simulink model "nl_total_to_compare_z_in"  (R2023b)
settings: Solver=VariableStepAuto  StartTime=0  StopTime=t(end)  RelTol=1e-9  AbsTol=1e-9
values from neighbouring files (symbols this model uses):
  cp_H2_coeff = [a_H2 b_H2 c_H2 d_H2]    [run_connect_all_sELY.m]
  cp_O2_coeff = [a_O2 b_O2 c_O2 d_O2]    [run_connect_all_sELY.m]
  eta_ACDC = 0.95    [run_connect_all_sELY.m]
  f1 = deg_model_eMTI.f1    [run_connect_all_sELY.m]
  f2 = deg_model_eMTI.f2    [run_connect_all_sELY.m]
  f3 = deg_model_eMTI.f3    [run_connect_all_sELY.m]
  f4 = deg_model_eMTI.f4    [run_connect_all_sELY.m]
  f5 = deg_model_eMTI.f5    [run_connect_all_sELY.m]
  F_farad = 96485    [run_connect_all_sELY.m]
  K_AW = 1/K_P    (= 2e-05)    [run_connect_all_sELY.m]
  K_I = 500    [run_connect_all_sELY.m]
  K_Ic = 0.01    [run_connect_all_sELY.m]
  K_max = P_cool_lim    (= 350000)    [run_connect_all_sELY.m]
  K_min = 0    [run_connect_all_sELY.m]
  K_P = 50000    [run_connect_all_sELY.m]
  M_H2 = 2.0159*1e-3    (= 0.0020159)    [run_connect_all_sELY.m]
  p_an = 29    [run_connect_all_sELY.m]
  p_BoP_prod = 0.05    [run_connect_all_sELY.m]
  P_BoP_sb = 7.1258e+03    (= 7125.8)    [run_connect_all_sELY.m]
  p_cat = 30    [run_connect_all_sELY.m]
  P_min_solve = 1e-3    (= 0.001)    [run_connect_all_sELY.m]
  R = 8.3145    [run_connect_all_sELY.m]    (also in DemoMTI_DHN_Pongau.m = 1/(2*kIns*pi) *log(0.18/0.0899) + 1/(2*2.4*pi)*log(2/0.18); DemoMTI_Discretized_Single_pipe.m = 1/(2*kIns*pi) *log(0.18/0.0899) + 1/(2*2.4*pi)*log(2/0.18); nine_bus_network.m = blkdiag(R,Rdq(:,:,i)))
  T_set = 273.15+60    (= 333.15)    [run_connect_all_sELY.m]
  T_std = 298.15    [run_connect_all_sELY.m]
  V_std = 1.23    [run_connect_all_sELY.m]
  x0 = [333.15, 331.1803, 0, 0, 7.4629e+06, 0]    [run_connect_all_sELY.m]    (also in DemoMTI_Boolean_Index_MTI.m = [0.5 0.0000]; DemoMTI_EKF.m = [1;-1;0.5]; DemoMTI_hybridSystemsTankExamples.m = 30; DemoMTI_MHE_VanDePol.m = randn((numOsc)*2,1))
undefined symbols (not defined in the file or in its folder): A_new, C_th, N_new, R_th, V_th, W_pump_heat

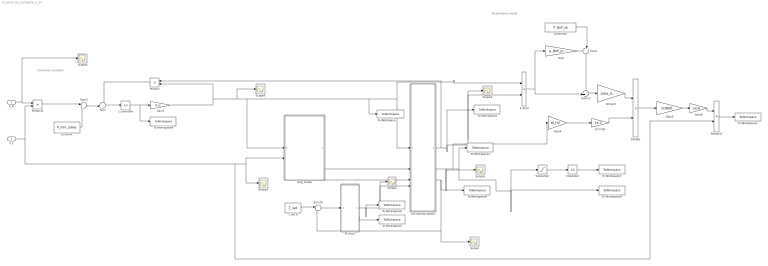
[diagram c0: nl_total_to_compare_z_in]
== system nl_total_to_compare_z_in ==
  note: Converter controller
  note: Performance model
  z_1 : Inport
  P_in : Inport  Port=2
  Constant : Constant  Value=P_min_solve
  Constant5 : Constant  Value=P_BoP_sb
  DC/AC2 : Gain  Gain=1/eta_ACDC
  Deg_model : Subsystem
  Divide1 : Product  Inputs=*/
  ELY without buffer : Subsystem
  Gain : Gain  Gain=p_BoP_prod
  Gain1 : Gain  Gain=K_Ic
  Gain4 : Gain  Gain=M_H2
  Gain5 : Gain  Gain=1/3600
  Gain6 : Gain  Gain=1e-6
  I_controller : Integrator  InitialCondition=x0(5)  LowerSaturationLimit=0
  Integrator : Integrator  InitialCondition=x0(6)
  PI_neu1 : Subsystem
  P_ELY2 : Product
  Product : Product
  Product1 : Product
  Product2 : Product
  Saturation : Saturate  UpperLimit=inf  LowerLimit=0
  Scope{,1..6} (7 alike) : Scope
  Sum : Sum  Inputs=-+|
  Sum1 : Sum  Inputs=++|
  Sum10 : Sum  Inputs=|-+
  Sum12 : Sum  Inputs=++|
  Sum2 : Sum  Inputs=|++
  T_set K : Constant  Value=T_set
  To Workspace : ToWorkspace  VariableName=I_in  SaveFormat=Timeseries  SampleTime=-1
  To Workspace1 : ToWorkspace  VariableName=e_H2_nl  SaveFormat=Timeseries  SampleTime=-1
  To Workspace2 : ToWorkspace  VariableName=V_ELY  SaveFormat=Timeseries  SampleTime=-1
  To Workspace3 : ToWorkspace  VariableName=n_H2  SaveFormat=Timeseries  SampleTime=-1
  To Workspace4 : ToWorkspace  VariableName=T_ELY  SaveFormat=Timeseries  SampleTime=-1
  To Workspace5 : ToWorkspace  VariableName=xQpi1  SaveFormat=Timeseries  SampleTime=-1
  To Workspace6 : ToWorkspace  VariableName=Q_cool  SaveFormat=Timeseries  SampleTime=-1
  To Workspace7 : ToWorkspace  VariableName=n_H2_sys_tot  SaveFormat=Timeseries  SampleTime=-1
  To Workspace8 : ToWorkspace  VariableName=n_H2_sys_flow  SaveFormat=Timeseries  SampleTime=-1
  To Workspace9 : ToWorkspace  VariableName=xI  SaveFormat=Timeseries  SampleTime=-1
  g in kg1 : Gain  Gain=1e-3
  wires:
  ELY without buffer/3(T_ely) -> To Workspace4/1, Sum10/2, Scope/1
  Gain1/1 -> Scope4/1, To Workspace/1, P_ELY2/1, ELY without buffer/1(I_in), Deg_model/1(I_in), Product/2
  Gain4/1 -> g in kg1/1
  g in kg1/1 -> Divide1/2
  P_ELY2/1 -> Sum12/2, Gain/1
  Gain5/1 -> Gain6/1
  Sum12/1 -> DC/AC2/1
  Constant5/1 -> Sum1/2
  DC/AC2/1 -> Divide1/1
  Divide1/1 -> Gain5/1
  Gain6/1 -> Product1/1
  Deg_model/1(V_act_deg) -> ELY without buffer/2(V_act_deg)
  Deg_model/2(R_ohm_deg) -> ELY without buffer/3(R_ohm_deg)
  z_1/1 -> Product2/2, Product1/2, Scope3/1, Deg_model/2(u_on_off)
  ELY without buffer/1(V_ELY) -> Scope2/1, P_ELY2/2, To Workspace2/1, Product/1
  Product/1 -> Sum/1
  P_in/1 -> Scope6/1, Product2/1
  T_set K/1 -> Sum10/1
  PI_neu1/2(state2) -> To Workspace5/1
  Sum10/1 -> PI_neu1/1(In1)
  PI_neu1/1(Q_cooling) -> To Workspace6/1, Scope1/1, ELY without buffer/4(Q_cool)
  Product1/1 -> To Workspace1/1
  Sum/1 -> I_controller/1
  I_controller/1 -> To Workspace9/1, Gain1/1
  Sum1/1 -> Sum12/1
  Gain/1 -> Sum1/1
  Product2/1 -> Sum2/1
  Sum2/1 -> Sum/2
  Constant/1 -> Sum2/2
  Integrator/1 -> To Workspace7/1
  ELY without buffer/2(n_H2) -> Scope5/1, To Workspace8/1, Saturation/1, To Workspace3/1, Gain4/1
  Saturation/1 -> Integrator/1

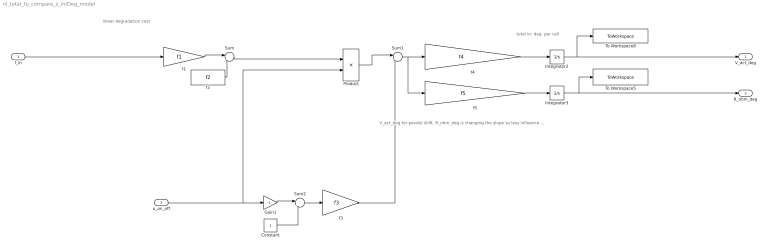
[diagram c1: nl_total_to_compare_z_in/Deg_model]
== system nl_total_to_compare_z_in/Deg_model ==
  note: linear degradation cost
  note: total irr. deg. per cell
  note: V_act_deg for paralel shift. R_ohm_deg is changing the slope so less influence in partial load.
  I_in : Inport
  u_on_off : Inport  Port=2
  Constant : Constant
  Gain1 : Gain  Gain=-1
  Integrator2 : Integrator  InitialCondition=x0(3)
  Integrator3 : Integrator  InitialCondition=x0(4)
  Product : Product
  Sum : Sum  Inputs=|++
  Sum1 : Sum  Inputs=|++
  Sum2 : Sum  Inputs=|++
  To Workspace5 : ToWorkspace  VariableName=R_ohm_deg  SaveFormat=Timeseries  SampleTime=-1
  To Workspace8 : ToWorkspace  VariableName=V_act_deg  SaveFormat=Timeseries  SampleTime=-1
  f1 : Gain  Gain=f1
  f2 : Constant  Value=f2
  f3 : Gain  Gain=f3
  f4 : Gain  Gain=f4
  f5 : Gain  Gain=f5
  V_act_deg : Outport
  R_ohm_deg : Outport  Port=2
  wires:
  f1/1 -> Sum/1
  f3/1 -> Sum1/2
  f2/1 -> Sum/2
  Sum1/1 -> f5/1, f4/1
  Integrator3/1 -> R_ohm_deg/1, To Workspace5/1
  I_in/1 -> f1/1
  Sum/1 -> Product/1
  f5/1 -> Integrator3/1
  Integrator2/1 -> V_act_deg/1, To Workspace8/1
  f4/1 -> Integrator2/1
  u_on_off/1 -> Product/2, Gain1/1
  Product/1 -> Sum1/1
  Gain1/1 -> Sum2/1
  Sum2/1 -> f3/1
  Constant/1 -> Sum2/2

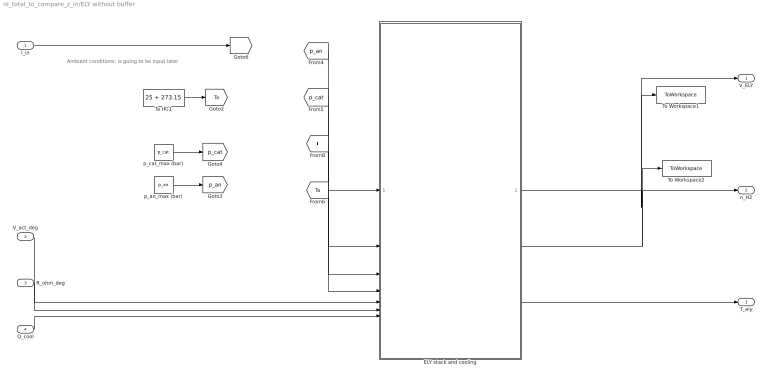
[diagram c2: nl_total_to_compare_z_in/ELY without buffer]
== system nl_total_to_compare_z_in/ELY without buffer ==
  note: Ambient conditions: is going to be input later
  I_in : Inport
  V_act_deg : Inport  Port=2
  R_ohm_deg : Inport  Port=3
  Q_cool : Inport  Port=4
  ELY stack and cooling : Subsystem
      mask init:
      | % for 400 A
      | %x0Temp1=333.1500;
      | %x0Temp2=3.329024438021895e+02;
      | %x0Qpi=5.618311056096404e+03;
      | %x0V_act=19.360033620504169;
      | 
      | %P_Q=-1662.44867463832; I_Q=-25.4752882159372;
  Ta (K)1 : Constant  Value=25 + 273.15
  To Workspace1 : ToWorkspace  VariableName=yVely  SaveFormat=Timeseries  SampleTime=-1
  To Workspace2 : ToWorkspace  VariableName=yH2ely  SaveFormat=Timeseries  SampleTime=-1
  p_an_max (bar) : Constant  Value=p_an
  p_cat_max (bar) : Constant  Value=p_cat
  V_ELY : Outport
  n_H2 : Outport  Port=2
  T_ely : Outport  Port=3
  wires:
  [p_an] -> ELY stack and cooling/1(p_an)
  V_act_deg/1 -> ELY stack and cooling/5(V_act_deg)
  I_in/1 -> [I]
  ELY stack and cooling/3(T_state1) -> T_ely/1
  R_ohm_deg/1 -> ELY stack and cooling/6(R_ohm_deg)
  p_an_max (bar)/1 -> [p_an]
  ELY stack and cooling/1(V_ELY (V)) -> V_ELY/1, To Workspace1/1
  Ta (K)1/1 -> [Ta]
  [Ta] -> ELY stack and cooling/4(Ta)
  p_cat_max (bar)/1 -> [p_cat]
  [p_cat] -> ELY stack and cooling/2(p_cat)
  [I] -> ELY stack and cooling/3(I)
  ELY stack and cooling/2(n_H2_tot) -> To Workspace2/1, n_H2/1
  Q_cool/1 -> ELY stack and cooling/7(Q_cool)

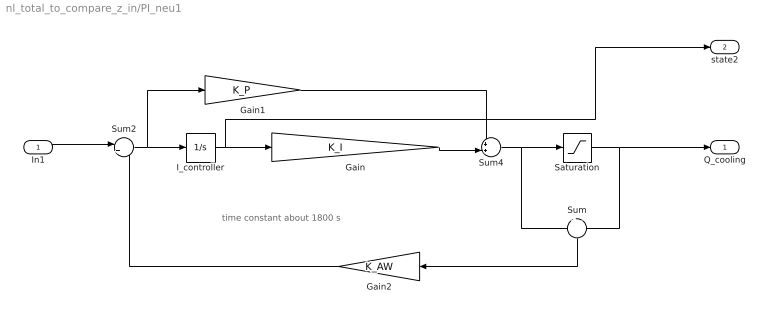
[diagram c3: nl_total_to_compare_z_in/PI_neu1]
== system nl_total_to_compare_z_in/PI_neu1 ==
  note: time constant about 1800 s
  In1 : Inport
  Gain : Gain  Gain=K_I
  Gain1 : Gain  Gain=K_P
  Gain2 : Gain  Gain=K_AW
  I_controller : Integrator  InitialCondition=x0(2)  LowerSaturationLimit=0
  Saturation : Saturate  UpperLimit=K_max  LowerLimit=K_min
  Sum : Sum  Inputs=+|-
  Sum2 : Sum  Inputs=|+-
  Sum4 : Sum  Inputs=++|
  Q_cooling : Outport
  state2 : Outport  Port=2
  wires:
  In1/1 -> Sum2/1
  Gain1/1 -> Sum4/1
  Sum4/1 -> Sum/1, Saturation/1
  Sum/1 -> Gain2/1
  Gain2/1 -> Sum2/2
  Saturation/1 -> Q_cooling/1, Sum/2
  Sum2/1 -> I_controller/1, Gain1/1
  I_controller/1 -> state2/1, Gain/1
  Gain/1 -> Sum4/2

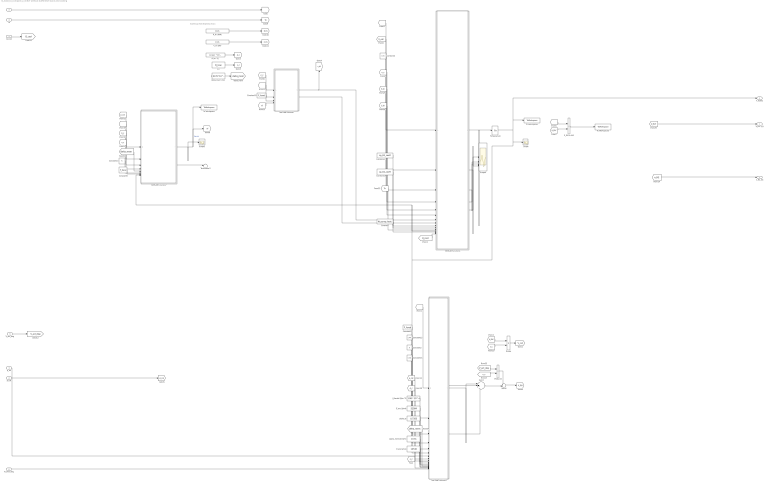
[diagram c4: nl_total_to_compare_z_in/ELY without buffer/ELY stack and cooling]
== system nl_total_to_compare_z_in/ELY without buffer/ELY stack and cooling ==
  note: Scaled up from Espinosa et al.:
  p_an : Inport
  p_cat : Inport  Port=2
  I : Inport  Port=3
  Ta : Inport  Port=4
  V_act_deg : Inport  Port=5
  R_ohm_deg : Inport  Port=6
  Q_cool : Inport  Port=7
  A (m^2) : Constant  Value="A_new  * 10^-4"
  C_th (J/K) : Constant  Value=C_th
  Constant : Constant  Value=W_pump_heat
  Constant10 : Constant  Value=R
  Constant13 : Constant  Value=F_farad
  Constant14 : Constant  Value=F_farad
  Constant15 : Constant  Value=T_std
  Constant16 : Constant  Value=V_std
  Constant17 : Constant  Value=cp_H2_coeff
  Constant18 : Constant  Value=cp_O2_coeff
  Constant2 : Constant  Value=R
  Constant4 : Constant  Value=V_th
  Constant9 : Constant  Value=F_farad
  Divide : Product  Inputs=*/
  E_exc (J/mol) : Constant  Value=52994
  E_pro (J/mol) : Constant  Value=10536
  MATLAB Function : MATLAB Function  TreatAsAtomicUnit=on
  MATLAB Function1 : MATLAB Function  TreatAsAtomicUnit=on
  MATLAB Function2 : MATLAB Function  TreatAsAtomicUnit=on
  MATLAB Function7 : MATLAB Function  TreatAsAtomicUnit=on
  P_ELY in W1 : Product
  Product2 : Product
  R_th (K/W) : Constant  Value=R_th
  Scope : Scope
  Scope2 : Scope
  Scope4 : Scope  NumInputPorts=5
  Sum3 : Sum  Inputs=|+++
  Sum5 : Sum  Inputs=++|
  Temperature : Integrator  InitialCondition=x0(1)
  Terminator3 : Terminator
  To Workspace : ToWorkspace  VariableName=nF  SaveFormat=Timeseries  SampleTime=-1
  To Workspace1 : ToWorkspace  VariableName=xTemp  SaveFormat=Timeseries  SampleTime=-1
  To Workspace3 : ToWorkspace  VariableName=P_ELY  SaveFormat=Timeseries  SampleTime=-1
  alpha_an : Constant  Value=0.7353
  delta_mem (m)1 : Constant  Value=0.0178 *10^-2
  i_0anstd (A/m^2) : Constant  Value=1.08 * 10^-4
  n_c : Constant  Value=N_new
  sigma_memstd (S/m) : Constant  Value=10.31
  V_ELY (V) : Outport
  n_H2_tot : Outport  Port=2
  T_state1 : Outport  Port=3
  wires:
  p_an/1 -> MATLAB Function2/7(p_an)
  p_cat/1 -> [p_cat]
  Constant14/1 -> MATLAB Function2/3(F)
  E_pro (J/mol)/1 -> MATLAB Function2/15(E_pro)
  [C_th] -> MATLAB Function1/6(C_th)
  [V_cell] -> MATLAB Function1/2(V_cell)
  MATLAB Function/1(n_H2) -> [n_H2], MATLAB Function1/7(n_H2)
  n_c/1 -> [n_c]
  MATLAB Function1/1(dTdt) -> Temperature/1
  i_0anstd (A/m^2)/1 -> MATLAB Function2/10(i_0anstd)
  [I] -> MATLAB Function1/1(I)
  alpha_an/1 -> MATLAB Function2/12(alpha_an)
  E_exc (J/mol)/1 -> MATLAB Function2/11(E_exc)
  [I] -> MATLAB Function2/1(I)
  [delta_mem] -> MATLAB Function2/13(delta_mem)
  [Ta] -> MATLAB Function1/11(Ta)
  Constant15/1 -> MATLAB Function2/4(T_std)
  Constant13/1 -> MATLAB Function/3(F)
  Constant17/1 -> MATLAB Function1/9(cp_coeff_H2)
  sigma_memstd (S/m)/1 -> MATLAB Function2/14(sigma_memstd)
  [A_c] -> MATLAB Function2/9(A)
  MATLAB Function/2(n_O2) -> MATLAB Function1/8(n_O2)
  Constant18/1 -> MATLAB Function1/10(cp_coeff_O2)
  [R_th] -> MATLAB Function1/5(R_th)
  [n_c] -> MATLAB Function/1(n_c)
  [n_c] -> MATLAB Function1/4(n_c)
  Constant4/1 -> MATLAB Function1/3(V_th)
  [I] -> MATLAB Function/2(I)
  Ta/1 -> [Ta]
  I/1 -> [I]
  P_ELY in W1/1 -> To Workspace3/1
  MATLAB Function2/3(V_act) -> Sum3/3
  MATLAB Function2/1(V_ocv) -> Sum3/1
  MATLAB Function2/2(V_ohm) -> Sum3/2
  [n_c] -> MATLAB Function2/16(n_c)
  [V_ELY] -> V_ELY (V)/1
  A (m^2)/1 -> [A_c]
  R_th (K/W)/1 -> [R_th]
  C_th (J/K)/1 -> [C_th]
  Constant2/1 -> MATLAB Function2/5(R)
  Constant16/1 -> MATLAB Function2/6(V_std)
  [V_ELY] -> P_ELY in W1/2
  [I] -> P_ELY in W1/1
  Divide/1 -> [V_cell]
  [V_ELY] -> Divide/1
  R_ohm_deg/1 -> MATLAB Function2/17(R_ohm_deg)
  [p_cat] -> MATLAB Function2/8(p_cat)
  delta_mem (m)1/1 -> [delta_mem]
  [n_c] -> Divide/2
  V_act_deg/1 -> [V_act_deg]
  [V_act_deg] -> Product2/1
  Sum5/1 -> [V_ELY]
  Sum3/1 -> Sum5/2
  [n_c] -> Product2/2
  Product2/1 -> Sum5/1
  [p_cat] -> MATLAB Function7/1(p_h2)
  [delta_mem] -> MATLAB Function7/5(delta_mem)
  [A_c] -> MATLAB Function7/3(A_cell)
  MATLAB Function7/1(eta_fara_h2) -> Scope2/1, To Workspace/1, [nf]  "Patrick"
  Temperature/1 -> To Workspace1/1, T_state1/1, Scope/1, MATLAB Function1/12(T), MATLAB Function7/8(T), MATLAB Function2/2(T)
  [I] -> MATLAB Function7/2(I)
  [n_c] -> MATLAB Function7/4(n_cell)
  MATLAB Function7/2(h2_o2) -> Terminator3/1
  Constant9/1 -> MATLAB Function7/7(F)
  Constant10/1 -> MATLAB Function7/6(R)
  [nf] -> MATLAB Function/4(nF)
  Q_cool/1 -> [Q_cool]
  [Q_cool] -> MATLAB Function1/14("Q_cooling ")
  MATLAB Function1/3(Q_loss) -> Scope4/2
  MATLAB Function1/4(sum_n_dh) -> Scope4/3
  MATLAB Function1/5(Q_cooling) -> Scope4/4
  MATLAB Function1/2(W_pemwe_heat) -> Scope4/1
  Constant/1 -> MATLAB Function1/13(W_pump_heat)
  [n_H2] -> n_H2_tot/1

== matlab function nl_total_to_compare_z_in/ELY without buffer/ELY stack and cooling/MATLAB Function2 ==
 function [V_ocv,V_ohm,V_act] = Electrochem_model(I,T,F,T_std,R,V_std,p_an,p_cat,A,i_0anstd,E_exc,...
    alpha_an,delta_mem,sigma_memstd,E_pro,n_c,R_ohm_deg)
%
%Electrochemical sub-model of electrolyzer for calculation of cell voltage
%
%(as long not other noted, inputs and outputs are scalar values)
%inputs:
% I         - DC current                        - A
% T         - cell temperature                  - K 
% F         - Faraday's constant                - C/mol
% T_std     - standard temperature              - K 
% R         - universal gas constant            - J/(mol K)
% V_std     - standard cell voltage             - V
% p_an      - anodic pressure                   - bar 
% p_cat     - cathodic pressure                 - bar 
% A         - Active catalyst area              - m^2
% i_0anstd  - electrode exchange current density anode standard - A/m^2
% (i_0anstd from Webster et al.)
% E_exc     - activation energy required for the electron transport in
% the anode electrode - J/mol
% alpha_an  - charge transfer coefficient anode - /
% delta_mem - membrane thickness                - m
% sigma_memstd - protonic conductivity          - S/m
% E_pro     - activation energy required for the proton transport in
% the membrane                                  - J/mol
% V_act     - activation overpotential          - V
% n_c       - number of cells                   - - 
%
%outputs:
% I_farad - Faraday current                     - A
% V_ocv - open circuit voltage                  - V
% V_ohm - ohmic voltage                         - V
% dVactdt - change of activation voltage        - V/s
%% ------------------------------------------------------------------------

i = I/A;                    % in A/m^2

p_an = p_an/1.01325;        %bar in atm
p_cat = p_cat/1.01325;      %bar in atm

%% ------------ open-circuit voltage --------------------------------------

V_rev = V_std - 0.0009*(T-T_std);

% Esp. Eq. (5)-(7)
p_H2O = 6.1078*10^-3*exp(17.2694*((T-273.15)/(T-34.85))); %in atm!!!
p_H2 = p_cat - p_H2O; %in atm
p_O2 = p_an - p_H2O; %in atm

%Durckabhängigkeit Ggw.-spannung
V_ocv_cell = V_rev + ((R*T)/(2*F))*(log((p_H2*p_O2^0.5)/p_H2O));
V_ocv = V_ocv_cell * n_c;
%% ------------activation overvoltage -------------------------------------
% Esp. Eq. (11)
i_0an = i_0anstd*exp(-(E_exc/R)*(1/T-1/T_std)); % A/m^2

%activation overpotential 
%Volmer-Butler-Equation (Esp. Eq. (10))
V_act = ((R*T)/(2*alpha_an*F))*asinh(i/(2*i_0an))*n_c;


%% ------------ohmic overvoltage-------------------------------------------
% Esp. Eq. (16)
sigma_mem = sigma_memstd*exp(-(E_pro/R)*(1/T-1/T_std)); % in S/m
% Esp. Eq. (14)
R_mem = delta_mem / sigma_mem; % m/(S/m) = m^2/S = Ohm m^2
%considering degradation
R_mem_tot = R_mem + R_ohm_deg;
% Esp. Eq. (13)
V_ohm = R_mem_tot * i *n_c; %total for whole stack (*n_c) / Ohm m^2 * A/m^2 = V

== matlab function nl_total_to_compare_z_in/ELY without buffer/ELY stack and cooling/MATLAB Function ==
function [n_H2,n_O2] = productionH2O2(n_c,I,F,nF)

%Hydrogen and oxygen prodcution of electrolyzer

%(as long not other noted, inputs and outputs are scalar values)
%inputs:
% n_c       - number of cells                   - /
% I         - DC current                        - A
% F         - Faraday's constant                - C/mol
% nF        - Faraday's efficiency              - /

%outputs:
% n_H2      - produced H2 stream                - mol/s
% n_O2      - produced O2 stream                - mol/s

%--------------------------------------------------------------------------

%h2_evo = I/2/F * n_cell; % mol/s
n_H2 = ((n_c*I)/(2*F))*nF;

%o2_evo = I/4/F * n_cell; % mol/s
n_O2 = n_H2/2;

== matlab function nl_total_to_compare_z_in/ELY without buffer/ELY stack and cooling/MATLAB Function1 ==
   function [dTdt,W_pemwe_heat,Q_loss,sum_n_dh,Q_cooling]= Thermal_model_T_DGL(I,V_cell,V_th,n_c,R_th,C_th,n_H2,...
    n_O2,cp_coeff_H2,cp_coeff_O2,Ta,T,W_pump_heat,Q_cooling)

%Thermal sub-model of electrolyzer for calculation of cell temperature

%(as long not other noted, inputs and outputs are scalar values)
%inputs:
% I         - DC current                        - A
% V_cell    - cell voltage                      - V
% V_th      - thermoneutral cell voltage        - V
% n_c       - number of cells                   - /
% R_th      - thermal resistance                - K/W
% C_th      - lumped thermal capacity           - J/K
% n_H2      - produced H2 stream                - mol/s 
% n_O2      - produced O2 stream                - mol/s
% cp_coeff_H2 [4x1] - heat hapacity coefficients H2 - for cp in J/ (mol K)
% cp_coeff_O2 [4x1] - heat hapacity coefficients O2 - for cp in J/ (mol K)
% Ta        - ambient temperature               - K
% T         - cell temperature                  - K 
% W_pump_heat - heat flow rate of pump          - W
% Q_cooling - heat flow rate of cooling         - W

%outputs:
%dTdt - change of cell temperature over time    - K/s
%---------------------Heat capacity----------------------------------------
a_H2 = cp_coeff_H2(1);
b_H2 = cp_coeff_H2(2);
c_H2 = cp_coeff_H2(3);
d_H2 = cp_coeff_H2(4);

a_O2 = cp_coeff_O2(1);
b_O2 = cp_coeff_O2(2);
c_O2 = cp_coeff_O2(3);
d_O2 = cp_coeff_O2(4);

cp_H2 = a_H2 + b_H2*T + c_H2*T^2 + d_H2*T^3; %HeatCapacity(T,a_H2,b_H2,c_H2,d_H2); 
cp_O2 = a_O2 + b_O2*T + c_O2*T^2 + d_O2*T^3; %HeatCapacity(T,a_O2,b_O2,c_O2,d_O2); 
%---------------------Reaktion heat----------------------------------------
% Eq. (18) Espinosa et al. 
W_pemwe_heat = ((V_cell - V_th)*I)*n_c;

%---------------------Heat losses------------------------------------------
%Eq. (22) Espinosa et al. 
Q_loss = 1/R_th*(T-Ta);

%---------------------Enthalpy streams-------------------------------------
% Eq. (23) Espinosa et al.
sum_n_dh = n_H2*cp_H2*(T-Ta) + n_O2*cp_O2*(T-Ta);

%---------------------toal diff. eq.---------------------------------------
% Eq. (17) Espinosa et al. 
dTdt = (W_pemwe_heat + W_pump_heat - Q_cooling - Q_loss - sum_n_dh)/C_th;

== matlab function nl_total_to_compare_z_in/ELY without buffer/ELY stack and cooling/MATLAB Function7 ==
function [eta_fara_h2, h2_o2] = faraday_efficiency_Patrick(p_h2,I, A_cell,n_cell,delta_mem,R,F,T)
%Crossover Model von Patrick Trinke
% inputs:
% p_h2   - hydrogen pressure        - in bar 
% I      - electrolyzer current     - in A
% A_cell - cross section of the studied PEM electrolyzer - in m^2
% n_cell - number of cells          - /
% delta_mem - membrane thickness    - m
% R - ideal gas constant            - J/(mol K)
% F - faraday constant              - As/mol 
% T - Temperature                   - K
% outputs: 
% eta_fara_h2 - faraday efficiency  - in /
% h2_o2  - H2 in O2                 - in in vol.%
%


%% Eingangparameter
% Kathodendruck
p_h2 = p_h2 * 1e5; % Pa


%% Parameter
% Diffusionskoeff:
% Dummy: D_h2 = 5e-9; % m²/s
% Dis Patrick, S. 110 Tab. A2, Eq. (A.6)
D_dsg_h2_T_0 = 4.9e-6; %m^2/s
E_h2 = 16.51e3; %J/mol
D_dsg_h2_T = D_dsg_h2_T_0 * exp(-E_h2/(R*T));
% Dis Patrick, S. 61 Eq. (6.9)
eps_ion = 1; % Ionomer fraction in the membrane Tab. 6.1 
eps_H2O = 0.42; %Tab. 4.2 = 0.37 / Tab. 5.1 = 0.42 / εH2O the water fraction within the ionomer,
tau_ion = 1.5; %Tab. 4.2 same in Tab. 1.5 / tortuosity of the ionomer channels
D_eff_dsg_h2 = ((eps_ion*eps_H2O)/tau_ion)*D_dsg_h2_T;

%D_eff_dsg_h2 = 5e-9; % m²/s

% Löslichkeitskonstante
%Dummy value: S_h2 = 7e-6; % mol/m³/Pa
% Dis Patrick, S. 110 Tab. A2, Eq. (A.7)
A_h2 = -48.1611;
B_h2 = 5528.45;
C_h2 = 16.8893;
S_h2 = 0.55*exp(A_h2+B_h2/T+C_h2*log(T/100)); %T in K / result in mol/m³/Pa

% Faradaykonstante
%F = 96485; % As/mol 

% Mass transfer coefficient
% Dis Patrick, S. 38 Fig. 4.5 / material dependent / chosen value
k_l = 3e-2; % m/s


%% Geometrische Werte
% Membrandicke
%delta_mem = 125e-6; % m
% Zellfläche (Grundfläche)
%A_cell = 0.5; % m²
% Zellanzahl
%n_cell = 50; % #

% Stackfläche 
A_stack = A_cell * n_cell; % m²


%% Berechnungen:

% produzierte Gasströme
o2_evo = I/4/F * n_cell; % mol/s
h2_evo = I/2/F * n_cell; % mol/s

% Übersättigte Wasserstoffkonzentration in der Kathode https://www.sciencedirect.com/science/article/abs/pii/S0360319917312971 
c_h2_super = (I/A_cell/2/F + k_l*p_h2*S_h2) / (k_l + D_eff_dsg_h2/delta_mem)  ; % mol/m³

% Crossoverfluss für den gesamten Stack
N_h2_cross_stack = D_eff_dsg_h2 * c_h2_super/delta_mem * A_stack; % mol/s

% H2 in O2
h2_o2 = N_h2_cross_stack / (N_h2_cross_stack + o2_evo) * 100; % in vol.%

% Faraday Wirkungsgrad
eta_fara_h2 = (1 - N_h2_cross_stack / h2_evo ); % in - 


% Notes: D, k_l und delta_mem sind potentielle Parameter die Altern
% könnten. D und S haben Temperaturabhängigkeiten
% Zur Crossover Theorie kannst du dir gerne das Paper angucken: https://www.sciencedirect.com/science/article/abs/pii/S0360319917312971
